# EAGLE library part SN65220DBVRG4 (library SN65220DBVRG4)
ESD Suppressors / TVS Diodes Sngl Port Transient Suppressor Source: Datasheet
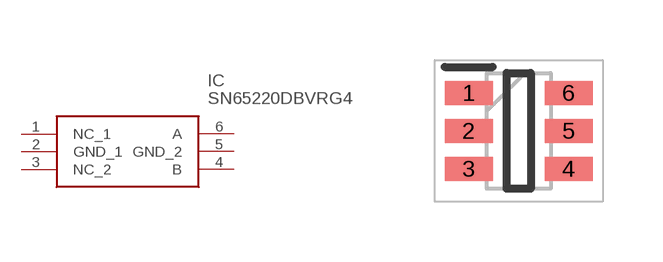
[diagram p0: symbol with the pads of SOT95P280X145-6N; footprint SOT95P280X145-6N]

Designator prefix IC

## SN65220DBVRG4 (Arrow_Part_Number: SN65220DBVRG4; Arrow_Price/Stock: https://www.arrow.com/en/products/sn65220dbvrg4/texas-instruments; Description: ESD Suppressors / TVS Diodes Sngl Port Transient Suppressor; Height: 1.45mm; Manufacturer_Name: Texas Instruments; Manufacturer_Part_Number: SN65220DBVRG4)  [SOT95P280X145-6N]
1  NC_1
2  GND_1  pwr
3  NC_2
4  B  in
5  GND_2  pwr
6  A  in

## Footprint SOT95P280X145-6N (pad centres in mm)
DBV (R-PDSO-G6)
smd 1.2 x 0.6: 1 -1.25,0.95; 2 -1.25,0; 3 -1.25,-0.95; 4 1.25,-0.95; 5 1.25,0; 6 1.25,0.95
